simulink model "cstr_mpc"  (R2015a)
settings: Solver=ode45  StartTime=0.0  StopTime=15  RelTol=1e-3
StopFcn:
  | plot_reactor
libraries: simulink x4

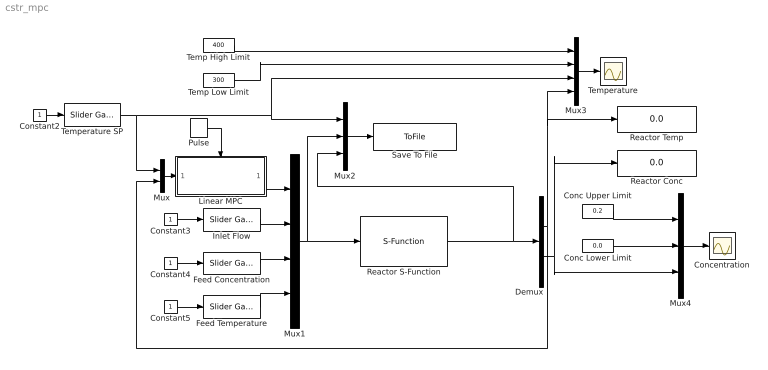
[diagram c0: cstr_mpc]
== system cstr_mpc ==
  Conc Lower Limit : Constant  Value=0.0
  Conc Upper Limit : Constant  Value=0.2
  Concentration : Scope
  Constant{2..5} (4 alike) : Constant
  Demux : Demux  Outputs=2
  Feed Concentration : simulink/Math Operations/Slider Gain  low=0  gain=1  high=1
  Feed Temperature : simulink/Math Operations/Slider Gain  low=300  gain=350  high=400
  Inlet Flow : simulink/Math Operations/Slider Gain  low=0  gain=100  high=200
  Linear MPC : Subsystem  TreatAsAtomicUnit=on
  Mux : Mux  Inputs=2
  Mux1 : Mux
  Mux2 : Mux  Inputs=3
  Mux3 : Mux
  Mux4 : Mux  Inputs=3
  Pulse : DiscretePulseGenerator  PulseType=Time based  Period=0.05  PulseWidth=5
  Reactor Conc : Display
  Reactor S-Function : S-Function  FunctionName=reactor
  Reactor Temp : Display
  Save To File : ToFile  Filename=data.mat  MatrixName=cstr  SampleTime=0.05
  Temp High Limit : Constant  Value=400
  Temp Low Limit : Constant  Value=300
  Temperature : Scope
  Temperature SP : simulink/Math Operations/Slider Gain  low=300  gain=350  high=400
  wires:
  Reactor S-Function/1 -> Mux2/3, Demux/1
  Constant3/1 -> Inlet Flow/1
  Mux2/1 -> Save To File/1
  Mux1/1 -> Mux2/2, Reactor S-Function/1
  Inlet Flow/1 -> Mux1/2
  Constant2/1 -> Temperature SP/1
  Temperature SP/1 -> Mux/1, Mux3/3, Mux2/1
  Demux/2 -> Mux4/3, Reactor Conc/1
  Constant4/1 -> Feed Concentration/1
  Feed Concentration/1 -> Mux1/3
  Constant5/1 -> Feed Temperature/1
  Feed Temperature/1 -> Mux1/4
  Demux/1 -> Mux/2, Mux3/4, Reactor Temp/1
  Temp High Limit/1 -> Mux3/1
  Temp Low Limit/1 -> Mux3/2
  Mux3/1 -> Temperature/1
  Conc Upper Limit/1 -> Mux4/1
  Conc Lower Limit/1 -> Mux4/2
  Mux4/1 -> Concentration/1
  Linear MPC/1(Out1) -> Mux1/1
  Pulse/1 -> Linear MPC/Trigger
  Mux/1 -> Linear MPC/1(In1)

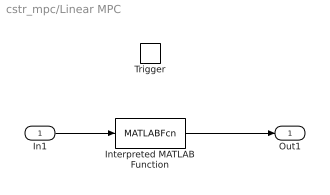
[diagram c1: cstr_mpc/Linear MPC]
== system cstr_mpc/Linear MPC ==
  In1 : Inport
  Trigger : TriggerPort
  Interpreted MATLAB Function : MATLABFcn  MATLABFcn=mpc
  Out1 : Outport
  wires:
  In1/1 -> Interpreted MATLAB Function/1
  Interpreted MATLAB Function/1 -> Out1/1
